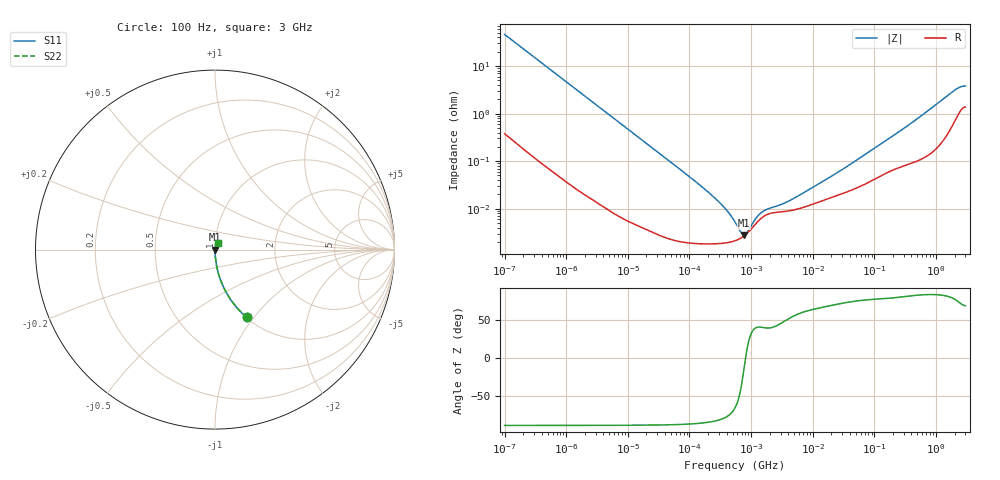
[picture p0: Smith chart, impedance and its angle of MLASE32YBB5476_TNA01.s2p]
! MLASE32YBB5476_TNA01  S-PARAMETER MODEL  ( Standard Model )
! Model Generated by TAIYO YUDEN Corporation (http://www.ty-top.com)
! Version 1.0
! TAIYO YUDEN Control No. 220601
! Copyright(c) 2011 TAIYO YUDEN CO.,LTD. All Rights Reserved.
! Product Description (link to TY-COMPAS)
! https://ds.yuden.co.jp/TYCOMPAS/or/detail?pn=MLASE32YBB5476MTNA01&u=M
! Products Name : Multilayer Ceramic Capacitors
! Characteristics :
!  Capacitance : 47 [uF] , Rated Voltage : 16 [V] , TCC : X5R
!  Case Size : 3.2 x 2.5 / 0.126 x 0.098 [mm/inch] , Thickness : 1.9 / 0.075 [mm/inch]
!  (Conditions: Temperature = 25 [degC] , DC Bias Voltage = 0 [V])
! External Node Assignments :
!  1  o---| |---o  2
! GND o---------o GND
! Frequency Range : 100Hz  -  3GHz  [ 401 STEP ]
# MHZ S RI R 50
! Freq[MHz].  S11 Real  S11 Imag  S21 Real  S21 Imag  S12 Real  S12 Imag  S22 Real  S22 Imag
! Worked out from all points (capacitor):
!   401 points, 100 Hz to 3 GHz, reference 50 ohm
!   read as one part in series: C = 34.5 uF near 109 Hz
!   lowest |Z| = 2.78 mohm at 772.9 kHz (marker M1)
!   series resonance near 814.3 kHz, so ESL is about 1.1 nH
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0.0001  0.1773 -0.3779  0.8227 0.3779  0.8227 0.3779  0.1773 -0.3779
0.000175  0.067 -0.2461  0.933 0.2461  0.933 0.2461  0.067 -0.2461
0.000348  0.0184 -0.1306  0.9816 0.1306  0.9816 0.1306  0.0184 -0.1306
0.000724  0.00461 -0.064  0.9954 0.064  0.9954 0.064  0.00461 -0.064
0.001788  0.000898 -0.0261  0.9991 0.0261  0.9991 0.0261  0.000898 -0.0261
0.031977  3e-05 -0.00148  1 0.00148  1 0.00148  3e-05 -0.00148
0.16412  1.83e-05 -0.000279  1 0.000279  1 0.000279  1.83e-05 -0.000279
0.2524  1.83e-05 -0.000172  1 0.000172  1 0.000172  1.83e-05 -0.000172
0.371814  1.9e-05 -0.000102  1 0.000102  1 0.000102  1.9e-05 -0.000102
0.423062  1.95e-05 -8.32e-05  1 8.32e-05  1 8.32e-05  1.95e-05 -8.32e-05
0.547723  2.12e-05 -4.83e-05  1 4.83e-05  1 4.83e-05  2.12e-05 -4.83e-05
0.772864  2.71e-05 -6.11e-06  1 6.11e-06  1 6.11e-06  2.71e-05 -6.11e-06
1.75092  7.39e-05 6.05e-05  0.9999 -6.05e-05  0.9999 -6.05e-05  7.39e-05 6.05e-05
2.079876  8.02e-05 6.62e-05  0.9999 -6.62e-05  0.9999 -6.62e-05  8.02e-05 6.62e-05
3.966702  8.95e-05 0.000111  0.9999 -0.000111  0.9999 -0.000111  8.95e-05 0.000111
9.794414  0.000123 0.000248  0.9999 -0.000248  0.9999 -0.000248  0.000123 0.000248
32.68714  0.000216 0.000682  0.9998 -0.000682  0.9998 -0.000682  0.000216 0.000682
175.1444  0.00061 0.00298  0.9994 -0.00298  0.9994 -0.00298  0.00061 0.00298
471.3361  0.00103 0.00734  0.999 -0.00734  0.999 -0.00734  0.00103 0.00734
1950.712  0.0072 0.0292  0.9928 -0.0292  0.9928 -0.0292  0.0072 0.0292
2419.119  0.0117 0.0335  0.9883 -0.0335  0.9883 -0.0335  0.0117 0.0335
3000  0.0148 0.0345  0.9852 -0.0345  0.9852 -0.0345  0.0148 0.0345
